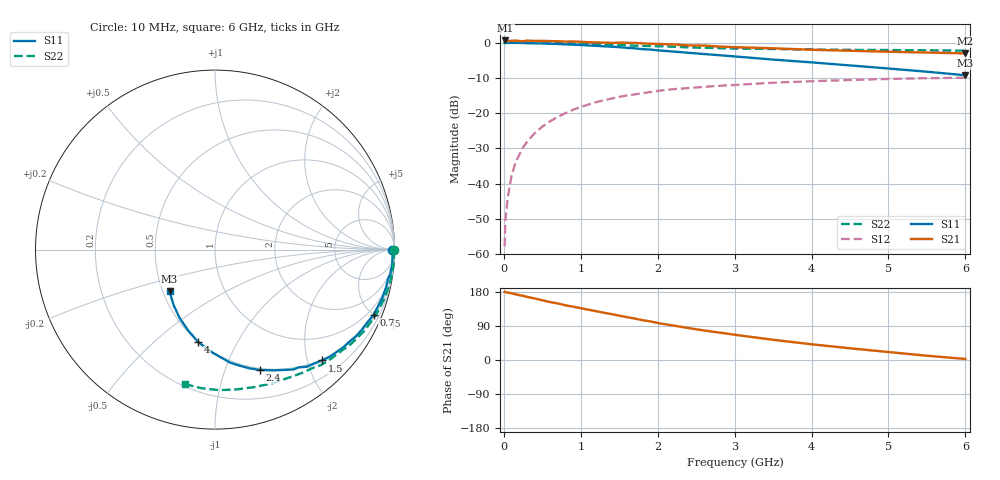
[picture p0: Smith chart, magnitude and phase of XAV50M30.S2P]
! SIEMENS Discrete & RF Semiconductors
! BFY180
! Si NPN RF Bipolar Junction Transistor in MICRO-X
! VCE = 0.5 V  IC = 0.3 mA
! Common Emitter S-Parameters:  May  1997
# GHz  S  MA  R  50
!  f  S11  S21  S12  S22
! GHz  MAG  ANG  MAG  ANG  MAG  ANG  MAG  ANG
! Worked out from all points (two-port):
!   36 points, 10 MHz to 6 GHz, reference 50 ohm
!   highest |S21| = 0.60 dB at 20 MHz (marker M1); lowest = -3.1 dB at 6 GHz (marker M2)
!   |S21| within 3 dB of the highest: start of sweep to 4.64 GHz
!   lowest |S11| = -9.3 dB at 6 GHz (marker M3), VSWR 2.05, Z = 27.1 - j14.3 ohm
!   |S11| at or under -10 dB: nowhere
!   |S22| runs from -2.3 to 0.0 dB; largest |S21 - S12| = 1.1
!   S11 on the Smith chart (normalised r, x): 10 MHz: open; 700 MHz: 0.60, -4.98; 1.5 GHz: 0.48, -2.28; 2.4 GHz: 0.48, -1.33; 4 GHz: 0.50, -0.71; 6 GHz: 0.54, -0.29
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0.01  0.9859 -0.2  1.038 180.0  0.0013 91.6  0.9981 -0.2
0.02  0.985 -0.5  1.071 179.1  0.003 95.0  0.9999 -0.5
0.05  0.9894 -1.6  1.053 177.9  0.0062 86.6  0.9978 -1.2
0.1  0.9895 -3.1  1.059 175.9  0.013 88.0  0.9982 -2.5
0.15  0.9918 -5.0  1.067 173.5  0.0196 85.7  0.9992 -3.6
0.2  0.9868 -6.4  1.052 171.1  0.0257 84.7  0.9984 -4.8
0.3  0.9778 -9.6  1.064 166.6  0.0389 81.8  0.9954 -7.2
0.4  0.976 -12.6  1.055 162.4  0.0518 79.4  0.9945 -9.5
0.7  0.9555 -22.4  1.044 149.3  0.0884 71.3  0.9808 -16.7
0.9  0.9328 -28.2  1.037 140.7  0.1116 65.8  0.9697 -21.3
1.1  0.9087 -34.1  1.012 132.7  0.1324 60.7  0.9548 -25.8
1.5  0.8596 -45.9  0.996 117.0  0.1698 51.1  0.924 -34.3
1.8  0.8059 -54.5  0.976 105.2  0.1916 44.9  0.8987 -40.1
2.2  0.7461 -64.4  0.942 91.0  0.2182 36.7  0.8728 -47.5
2.4  0.7159 -69.5  0.911 84.3  0.2263 33.3  0.8536 -50.8
2.6  0.6877 -74.0  0.907 78.0  0.2354 30.2  0.8445 -53.8
3  0.6358 -82.3  0.861 66.7  0.2504 24.0  0.8235 -60.0
3.5  0.5738 -91.5  0.829 53.3  0.2697 17.8  0.8101 -67.0
4  0.5237 -100.3  0.79 41.5  0.2829 11.3  0.7965 -74.2
4.5  0.474 -108.5  0.765 30.9  0.2948 5.3  0.7881 -81.3
5.5  0.3859 -126.7  0.722 11.3  0.3125 -6.1  0.7759 -95.6
6  0.3438 -137.5  0.702 2.7  0.3178 -11.8  0.768 -102.7
